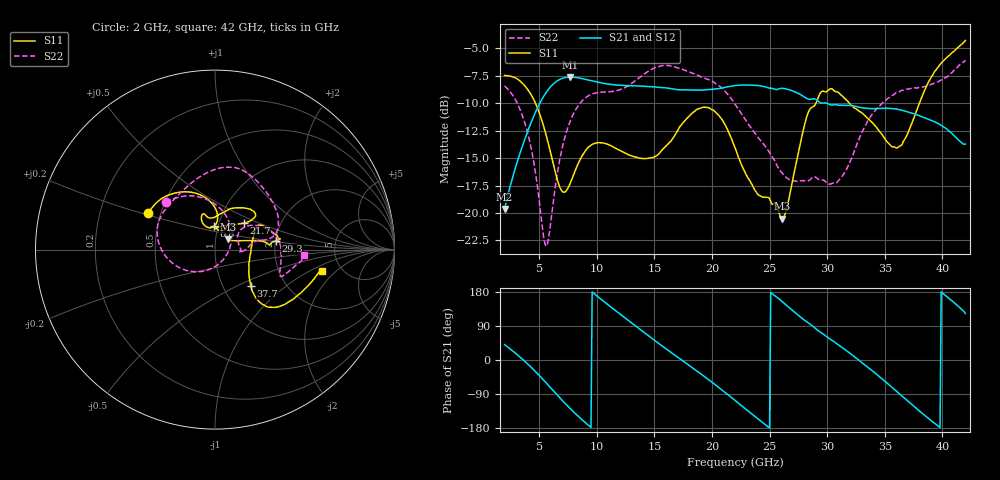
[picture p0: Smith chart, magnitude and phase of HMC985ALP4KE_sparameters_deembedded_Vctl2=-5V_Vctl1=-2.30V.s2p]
!s2p File: Measurements: S11, S21, S12, S22
# GHz S dB R 50.0
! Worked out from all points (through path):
!   401 points, 2 GHz to 42 GHz, reference 50 ohm
!   highest |S21| = -7.62 dB at 7.7 GHz (marker M1); lowest = -19.6 dB at 2 GHz (marker M2)
!   lowest |S11| = -20.5 dB at 26.1 GHz (marker M3), VSWR 1.21, Z = 57.5 + j6.78 ohm
!   |S11| at or under -10 dB: 4.677 GHz to 29.03 GHz (24.35 GHz wide, 144 % of centre); 31.93 GHz to 38 GHz (6.079 GHz wide, 17.4 % of centre)
!   |S22| runs from -23.0 to -6.1 dB; largest |S21 - S12| = 0.00051
!   S11 on the Smith chart (normalised r, x): 2 GHz: 0.43, +0.21; 6.8 GHz: 0.96, +0.25; 21.7 GHz: 1.31, +0.41; 29.3 GHz: 2.01, +0.22; 37.7 GHz: 1.35, -0.60; 42 GHz: 3.57, -1.37
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2  -7.47 151.5  -19.62 40.6  -19.63 40.6  -8.43 136.2
4  -8.74 118.3  -12.57 -10.4  -12.57 -10.4  -12.70 83.1
5.6  -12.89 89.1  -9.03 -60.2  -9.04 -60.2  -23.02 -33.1
6.8  -17.67 92.0  -7.83 -100.1  -7.83 -100.1  -15.05 -136.3
7.7  -17.28 111.0  -7.62 -128.4  -7.62 -128.4  -11.62 -167.1
8.7  -14.85 114.5  -7.75 -157.0  -7.75 -157.0  -9.81 170.0
10.3  -13.60 108.0  -8.14 162.0  -8.14 162.0  -9.00 146.6
12.3  -14.44 103.8  -8.38 114.6  -8.38 114.6  -8.65 121.7
15.4  -14.60 87.8  -8.57 43.1  -8.57 43.2  -6.64 80.8
18.3  -10.90 54.2  -8.80 -20.4  -8.80 -20.4  -7.27 50.7
21.7  -13.24 42.7  -8.44 -99.2  -8.45 -99.2  -9.61 12.5
22  -14.05 46.4  -8.39 -106.6  -8.40 -106.6  -10.07 11.5
24.1  -18.41 87.7  -8.40 -157.9  -8.40 -157.9  -13.24 11.0
26.1  -20.53 38.4  -8.64 154.1  -8.64 154.1  -16.38 -3.8
28.7  -10.35 4.7  -9.61 90.7  -9.62 90.7  -16.77 -2.5
29.3  -9.29 8.0  -9.88 75.6  -9.89 75.7  -16.97 1.0
30.9  -8.98 12.5  -10.16 41.5  -10.17 41.6  -17.16 25.1
32.4  -10.46 25.5  -10.27 7.8  -10.27 7.9  -14.26 37.6
35.4  -13.72 6.6  -10.46 -66.2  -10.46 -66.1  -9.48 15.6
37.7  -10.88 -45.7  -11.02 -126.5  -11.02 -126.4  -8.60 -6.2
39.7  -6.60 -43.3  -11.88 -175.9  -11.88 -175.9  -8.00 -22.3
42  -4.28 -11.4  -13.72 122.6  -13.73 122.6  -6.08 -3.6
